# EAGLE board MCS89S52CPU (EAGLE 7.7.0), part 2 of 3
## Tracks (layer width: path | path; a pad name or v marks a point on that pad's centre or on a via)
/CSEX  (via drill 0.61)
  Top 0.254: IC10.1 11.89,57.15 15.54,53.49 v18.06,53.49 | v31.09,50.75 31.09,49.38 v31.77,48.69 31.77,47.78 29.26,45.26 29.26,37.95 31.32,35.89 31.77,35.89 37.95,29.72 v40.23,29.72 | v34.98,50.98 34.98,55.32 40.46,60.81 IC14.20 | v118.87,15.09 117.73,13.95 v115.21,13.95 | v102.87,10.29 101.5,10.29 97.84,6.63 96.01,6.63 95.1,7.54 v95.1,10.29 | v88.01,12.8 86.64,14.17 83.21,14.17 75.44,21.95 75.44,23.32 74.52,24.23 72.69,24.23 v71.09,25.83 | v59.66,29.03 55.78,29.03 55.09,29.72 v43.2,29.72
  Bottom 0.254: v18.06,53.49 23.09,53.49 24.69,51.89 29.95,51.89 v31.09,50.75 | v31.77,48.69 32.69,48.69 v34.98,50.98 | v118.87,15.09 124.36,15.09 IC4.8 | v115.21,13.95 111.56,10.29 v102.87,10.29 | v95.1,10.29 90.53,10.29 v88.01,12.8 | v71.09,25.83 70.41,25.83 67.21,29.03 v59.66,29.03 | v40.23,29.72 v43.2,29.72
ADR0  (via drill 0.61)
  Top 0.254: v90.3,77.04 88.01,77.04 85.95,74.98 v82.07,74.98 | v71.55,68.58 71.55,64.69 72.01,64.24 72.01,61.95 68.58,58.52 IC2.10 | SV1.9 28.12,97.61 28.12,95.33 SV3.9 28.12,95.1 28.12,83.9 v30.86,81.15 | 39.09,56.46 40.01,57.38 45.95,57.38 IC3.10 | 39.09,56.46 v36.58,53.95 | v26.52,18.29 26.52,12.8 IC11.9 | v14.4,41.38 14.4,42.06 15.32,42.98 17.83,42.98 20.8,45.95 20.8,54.18 24.92,58.29 25.38,58.29 IC14.10 | v34.52,77.5 34.52,68.12 38.86,63.78 38.86,62.87 37.95,61.95 v37.26,61.95 | 39.09,56.46 v38.41,57.15
  Bottom 0.254: IC8.19 90.3,78.87 v90.3,77.04 | v82.07,74.98 78.41,71.32 77.95,71.32 76.35,69.72 72.69,69.72 v71.55,68.58 | v36.58,53.95 34.75,53.95 33.6,55.09 30.18,55.09 29.95,54.86 24.23,54.86 23.55,55.55 23.55,56.46 25.38,58.29 IC14.10 | v26.52,18.29 18.06,26.75 18.06,30.63 14.4,34.29 v14.4,41.38 | v34.52,77.5 v30.86,81.15 | v37.26,61.95 37.26,61.49 38.63,60.12 38.63,59.21 38.41,58.98 v38.41,57.15 | IC2.10 68.58,58.29 63.78,58.29 62.64,57.15 57.38,57.15 56.24,58.29 47.09,58.29 IC3.10
ADR1  (via drill 0.61)
  Top 0.254: v89.38,72.69 89.38,64.01 89.84,63.55 89.84,62.64 86.87,59.66 v81.38,59.66 | SV1.10 30.63,97.61 30.63,95.33 SV3.10 30.4,95.1 v30.4,83.44 | v24.23,18.97 24.23,12.8 IC11.8 | v13.49,40.46 13.49,41.83 15.09,43.43 17.6,43.43 20.34,46.18 20.34,55.78 25.38,60.81 IC14.9 | v28.12,81.15 28.12,66.52 26.29,64.69 24.46,64.69 23.55,63.78 v23.55,62.64 | v44.35,62.87 46.18,61.04 46.86,61.04 IC3.9
  Bottom 0.254: v89.38,72.69 89.38,82.75 92.58,85.95 100.36,85.95 101.5,84.81 101.5,82.75 100.81,82.07 99.9,82.07 98.3,83.67 97.84,83.67 IC8.18 | v81.38,59.66 79.55,59.66 78.87,58.98 77.04,58.98 75.21,60.81 68.58,60.81 | 68.58,60.81 64.92,60.81 63.78,59.66 61.72,59.66 61.27,60.12 49.15,60.12 48.46,60.81 47.09,60.81 IC3.9 | 68.58,60.81 IC2.9 | v24.23,18.97 24.23,19.89 17.6,26.52 17.6,30.4 13.49,34.52 v13.49,40.46 | v28.12,81.15 v30.4,83.44 | v23.55,62.64 25.38,60.81 IC14.9 25.6,60.81 30.63,60.81 31.32,60.12 33.38,60.12 37.95,64.69 41.6,64.69 43.43,62.87 v44.35,62.87
ADR2  (via drill 0.61)
  Top 0.254: v11.2,72.01 11.2,71.32 9.83,69.95 7.77,69.95 7.09,70.64 7.09,79.55 8.69,81.15 IC9.1 | v116.81,77.72 116.81,70.64 113.61,67.44 113.61,66.29 114.07,65.84 114.07,59.89 112.7,58.52 109.04,58.52 108.36,59.21 97.38,59.21 96.24,60.35 v96.24,62.64 | v86.41,66.52 v88.24,66.52 | v37.95,63.32 v34.52,63.32
  Bottom 0.254: v11.2,72.01 11.89,72.01 13.26,70.64 13.26,69.72 15.54,67.44 19.2,67.44 23.09,63.55 25.38,63.55 IC14.8 25.6,63.32 v34.52,63.32 | v116.81,77.72 116.81,80.01 115.9,80.92 98.53,80.92 96.7,82.75 96.7,84.81 97.38,85.5 98.53,85.5 100.13,83.9 IC8.17 | v96.24,62.64 95.1,62.64 93.73,64.01 93.73,65.84 93.04,66.52 v88.24,66.52 | v86.41,66.52 85.04,66.52 84.35,67.21 82.3,67.21 77.95,62.87 69.04,62.87 68.58,63.32 IC2.8 68.58,63.55 67.44,64.69 61.72,64.69 61.49,64.92 49.38,64.92 48.01,63.55 47.09,63.55 IC3.8 46.86,63.32 45.49,61.95 40.01,61.95 38.63,63.32 v37.95,63.32
ADR3  (via drill 0.61)
  Top 0.254: 11.2,76.35 8.91,78.64 IC9.2 | v11.2,74.07 11.2,76.35 | v79.55,76.58 82.98,80.01 84.35,80.01 84.81,80.47 99.21,80.47 102.41,83.67 102.87,83.67 IC8.16 | v66.98,70.41 66.98,69.49 66.75,69.27 66.75,67.89 68.58,66.06 IC2.7 68.58,65.84 66.29,63.55 66.29,56.69 65.61,56.01 v65.61,54.86 | v50.06,51.21 50.29,51.44 50.29,62.18 48.92,63.55 48.92,64.01 47.09,65.84 IC3.7 47.09,66.06 48.69,67.67 48.69,69.27 48.46,69.49 48.46,82.07 47.32,83.21 v40.23,83.21 | v14.86,80.01 11.2,76.35
  Bottom 0.254: v11.2,74.07 15.54,69.72 19.43,69.72 23.09,66.06 25.38,66.06 IC14.7 | v79.55,76.58 79.55,73.61 76.12,70.18 69.49,70.18 69.27,69.95 67.44,69.95 v66.98,70.41 | v50.06,51.21 51.44,51.21 51.89,51.66 61.27,51.66 61.72,52.12 62.87,52.12 v65.61,54.86 | v14.86,80.01 28.35,80.01 30.4,82.07 32.23,82.07 35.2,79.1 36.12,79.1 v40.23,83.21
ADR4  (via drill 0.61)
  Top 0.254: v23.55,72.24 23.55,70.87 25.38,69.04 25.38,68.58 IC14.6 | IC3.6 45.26,68.58 v44.35,69.49 | v85.5,73.61 84.35,72.47 83.44,72.47 80.7,69.72 80.7,67.89 v81.15,67.44 | v71.09,63.78 71.09,66.06 IC2.6 | v58.75,69.49 v56.92,67.67
  Bottom 0.254: v23.55,72.24 22.86,72.24 20.8,74.3 18.06,74.3 17.14,75.21 13.49,75.21 12.57,76.12 8.91,76.12 IC9.3 | v44.35,69.49 41.83,69.49 41.6,69.72 36.58,69.72 35.43,68.58 IC14.6 | v85.5,73.61 88.01,76.12 88.01,85.27 90.07,87.33 102.18,87.33 104.47,85.04 104.47,84.81 105.39,83.9 IC8.15 | v81.15,67.44 78.18,67.44 74.52,63.78 v71.09,63.78 | IC3.6 50.98,68.58 51.89,67.67 v56.92,67.67 | v58.75,69.49 61.27,69.49 61.72,69.95 66.06,69.95 67.44,68.58 IC2.6
ADR5  (via drill 0.61)
  Top 0.254: v86.87,87.78 86.18,87.78 v84.35,85.95 | v71.32,88.92 70.18,90.07 52.35,90.07 v49.61,92.81 | v36.8,90.3 36.8,85.72 29.03,77.95 v29.03,74.75 | v38.41,75.44 36.8,75.44 v36.58,75.67
  Bottom 0.254: IC2.5 68.58,71.32 65.61,71.32 64.47,72.47 61.72,72.47 60.35,71.09 47.09,71.09 IC3.5 46.86,71.32 46.18,71.32 42.29,75.21 38.63,75.21 v38.41,75.44 | IC9.6 8.69,68.58 8.69,69.04 7.09,70.64 7.09,74.07 8,74.98 13.03,74.98 15.77,72.24 22.17,72.24 23.09,71.32 25.38,71.32 IC14.5 v29.03,74.75 29.95,75.67 v36.58,75.67 | v86.87,87.78 103.56,87.78 107.44,83.9 107.9,83.9 IC8.14 | v84.35,85.95 83.67,85.95 82.3,87.33 76.12,87.33 72.69,90.75 71.78,90.75 71.32,90.3 v71.32,88.92 | v49.61,92.81 49.61,92.13 47.32,89.84 37.26,89.84 v36.8,90.3
ADR6  (via drill 0.61)
  Top 0.254: 11.66,68.81 14.86,72.01 14.86,74.3 15.77,75.21 v19.2,75.21 | v128.7,86.18 v123.67,86.18 | v122.99,36.8 113.39,36.8 108.36,41.83 104.01,41.83 100.36,38.18 v95.78,38.18 | v84.35,42.98 80.92,42.98 79.78,41.83 v78.87,41.83 | v72.69,47.09 61.72,47.09 56.01,52.81 56.01,56.69 | 56.01,56.69 56.01,69.27 57.61,70.87 | 57.61,70.87 61.72,74.98 67.44,74.98 68.58,73.84 IC2.4 | 57.61,70.87 v56.46,72.01 | v13.72,66.75 11.66,68.81 | 56.01,56.69 v56.46,56.69 | 11.66,68.81 v11.43,68.58
  Bottom 0.254: v11.43,68.58 11.43,57.61 8.91,55.09 8.91,54.63 IC10.2 | v19.2,75.21 24,75.21 25.38,73.84 IC14.4 | v123.67,86.18 122.99,86.87 113.16,86.87 110.64,84.35 110.64,83.9 IC8.13 | v128.7,86.18 131.44,86.18 137.16,80.47 152.93,80.47 154.99,78.41 154.99,72.01 155.45,71.55 155.45,46.41 149.73,40.69 149.73,37.72 144.47,32.46 126.64,32.46 122.99,36.12 v122.99,36.8 | v95.78,38.18 94.87,37.26 90.07,37.26 v84.35,42.98 | v78.87,41.83 77.95,41.83 v72.69,47.09 | v56.46,72.01 52.12,72.01 50.52,73.61 47.09,73.61 IC3.4 | v13.72,66.75 13.72,62.18 18.29,57.61 18.29,56.69 18.06,56.46 18.06,55.55 18.52,55.09 19.89,55.09 24.23,59.44 30.63,59.44 34.75,55.32 39.09,55.32 39.55,54.86 44.12,54.86 46.41,57.15 56.01,57.15 v56.46,56.69
ADR7  (via drill 0.61)
  Top 0.254: v45.72,79.78 45.72,78.18 46.86,77.04 46.86,76.35 IC3.3 | v126.87,73.61 v124.13,76.35 | v126.87,66.98 131.9,61.95 131.9,59.89 127.1,55.09 v119.1,55.09 | v114.53,31.55 113.84,31.55 110.87,28.57 110.87,24.92 109.96,24 108.13,24 107.21,23.09 v107.21,21.95 | v52.12,17.83 v59.66,17.83 | v11.66,45.72 11.66,46.63 8.91,49.38 IC10.4
  Bottom 0.254: IC2.3 68.58,76.81 62.87,82.53 61.04,82.53 56.92,78.41 55.55,78.41 53.95,80.01 46.41,80.01 46.18,79.78 v45.72,79.78 39.09,86.41 39.09,87.1 38.18,88.01 21.03,88.01 13.95,80.92 13.95,77.27 | 13.95,77.27 24.46,77.27 25.38,76.35 IC14.3 | 13.95,77.27 7.77,77.27 5.03,74.52 5.03,67.67 7.77,64.92 9.6,64.92 10.74,63.78 10.74,63.09 7.09,59.44 7.09,51.66 8.69,50.06 8.69,49.61 IC10.4 | v124.13,76.35 124.13,79.32 119.56,83.9 118.42,83.9 116.36,85.95 114.76,85.95 113.16,84.35 113.16,83.9 IC8.12 | v126.87,66.98 v126.87,73.61 | v119.1,55.09 119.1,44.58 114.53,40.01 v114.53,31.55 | v107.21,21.95 105.39,21.95 102.41,18.97 97.38,18.97 94.64,16.23 84.81,16.23 78.87,10.29 75.21,10.29 69.27,16.23 64.24,16.23 62.64,17.83 v59.66,17.83 | v52.12,17.83 51.66,17.83 50.06,16.23 25.6,16.23 21.03,20.8 21.03,21.26 15.09,27.2 15.09,32.23 11.66,35.66 v11.66,45.72
ADR8  (via drill 0.61)
  Top 0.254: SV3.13 38.18,95.33 38.18,97.61 SV1.13 | v18.97,56.01 19.43,55.55 19.43,50.29 17.6,48.46 15.77,48.46 11.89,44.58 8.91,44.58 IC10.6 | v37.72,59.66 37.72,60.12 40.01,62.41 41.83,62.41 42.29,62.87 v42.29,67.21 42.29,72.01 IC14.25 40.69,73.84 42.52,75.67 v42.52,80.47 | v58.29,67.67 59.66,69.04 59.66,70.41 62.18,72.92 62.18,73.61 IC3.25 | v38.18,86.64 38.18,87.55 | 38.18,87.55 v38.18,90.75 | v80.92,92.35 76.81,92.35 72.01,87.55 67.89,87.55 67.44,88.01 53.26,88.01 v52.81,87.55 | 38.18,87.55 v40.01,87.55
  Bottom 0.254: IC1.21 140.82,61.04 135.79,66.06 116.59,66.06 112.7,69.95 87.55,69.95 83.9,73.61 IC2.25 83.9,73.84 83.9,74.52 87.55,78.18 87.55,85.72 v80.92,92.35 | v18.97,56.01 20.12,56.01 24,59.89 30.86,59.89 31.09,59.66 v37.72,59.66 | v58.29,67.67 57.38,66.75 48.01,66.75 47.55,67.21 v42.29,67.21 | v38.18,90.75 38.18,95.1 SV3.13 | v38.18,86.64 42.52,82.3 v42.52,80.47 | v52.81,87.55 50.29,87.55 49.84,88.01 40.46,88.01 v40.01,87.55
ADR9  (via drill 0.61)
  Top 0.254: v126.64,56.92 103.56,56.92 v102.64,56.01 | v95.78,50.98 v97.61,50.98 | v88.7,53.26 88.7,54.86 90.3,56.46 90.3,58.29 89.84,58.75 89.84,61.27 90.75,62.18 90.75,66.29 92.58,68.12 92.58,71.55 90.53,73.61 86.87,73.61 84.58,71.32 83.9,71.32 IC2.24 | SV1.14 40.69,97.61 40.69,95.33 SV3.14 40.69,95.1 40.69,91.9 v45.49,87.1 | v22.63,54.41 21.26,53.03 21.26,44.58 17.6,40.92 15.77,40.92 14.4,39.55 8.91,39.55 IC10.8 | v30.63,54.18 30.63,65.15 31.77,66.29 v31.77,69.49 | v60.12,67.67 60.12,69.04 62.18,71.09 IC3.24 | v45.26,81.61 45.26,80.7 44.35,79.78 v44.35,70.87 45.26,69.95 47.32,69.95 48.23,69.04 48.23,68.12 47.32,67.21 46.41,67.21 v45.26,66.06 46.63,64.69 47.55,64.69 48.23,64.01 48.23,63.55 48.69,63.09 v48.69,50.75 | v89.61,45.03 89.61,37.72 87.55,35.66 87.55,34.98 82.98,30.4 77.5,30.4 v75.67,28.57 | v48.23,38.18 46.18,38.18 v45.72,38.63
  Bottom 0.254: v126.64,56.92 129.39,59.66 129.39,61.72 130.3,62.64 136.7,62.64 138.3,61.04 IC1.22 | v97.61,50.98 v102.64,56.01 | 94.87,50.98 v95.78,50.98 | 94.87,50.98 94.41,51.44 90.98,51.44 89.15,53.26 v88.7,53.26 | v22.63,54.41 30.4,54.41 v30.63,54.18 | v31.77,69.49 35.66,69.49 37.26,71.09 40.46,71.09 IC14.24 40.69,71.09 40.92,70.87 v44.35,70.87 | v60.12,67.67 57.84,65.38 48.01,65.38 47.32,64.69 46.63,64.69 v45.26,66.06 | v45.49,87.1 45.49,81.84 v45.26,81.61 | 94.87,50.98 94.87,50.06 92.81,48.01 92.13,48.01 89.61,45.49 v89.61,45.03 | v75.67,28.57 75.21,28.57 74.3,29.49 72.47,29.49 67.67,34.29 52.12,34.29 v48.23,38.18 | v45.72,38.63 45.72,48.69 46.63,49.61 47.55,49.61 v48.69,50.75
ADR10  (via drill 0.61)
  Top 0.254: IC14.21 40.46,63.32 40.01,63.32 34.06,57.38 v34.06,43.66 34.06,43.2 34.98,42.29 36.58,42.29 40.23,45.95 48.69,45.95 50.29,47.55 v50.29,48.69 | SV1.15 43.2,97.61 43.2,95.33 SV3.15 43.2,95.1 43.2,92.81 47.32,88.7 47.32,84.58 49.84,82.07 49.84,75.89 50.29,75.44 50.29,64.24 v50.06,64.01 | v95.78,54.63 96.24,54.18 126.87,54.18 132.36,59.66 132.36,62.18 132.82,62.64 134.19,62.64 135.79,61.04 IC1.23 | v52.35,63.09 v52.35,50.75
  Bottom 0.254: IC10.11 23.77,34.29 31.77,42.29 32.69,42.29 v34.06,43.66 | v95.78,54.63 92.58,54.63 91.44,53.49 90.53,53.49 85.5,58.52 85.5,61.72 83.9,63.32 IC2.21 83.67,63.32 81.15,63.32 80.01,62.18 68.12,62.18 66.98,63.32 62.41,63.32 IC3.21 61.72,64.01 52.35,64.01 | 52.35,64.01 v50.06,64.01 | v52.35,50.75 v50.29,48.69 | 52.35,64.01 v52.35,63.09
ADR11  (via drill 0.61)
  Top 0.254: v28.35,40.69 28.35,41.38 28.8,41.83 28.8,45.49 30.18,46.86 30.18,52.35 31.77,53.95 v31.77,61.04 | SV1.16 SV3.16 45.72,95.1 51.89,88.92 v69.95,88.92 | v114.07,74.52 114.07,76.81 115.9,78.64 120.47,78.64 136.93,62.18 136.93,59.89 136.25,59.21 135.56,59.21 133.96,60.81 133.5,60.81 IC1.24 | v88.01,70.87 86.18,70.87 83.9,68.58 IC2.23 | v74.98,82.3 75.67,82.3 76.81,83.44 v77.27,83.44 | v77.95,75.21 77.95,74.75 77.5,74.3 77.5,69.49 v78.64,68.35
  Bottom 0.254: v28.35,40.69 27.2,39.55 16.69,39.55 IC10.13 | v31.77,61.04 33.6,61.04 38.86,66.29 38.86,66.98 40.46,68.58 IC14.23 44.81,68.58 46.18,69.95 50.29,69.95 51.66,68.58 IC3.23 63.09,68.58 66.52,65.15 67.67,65.15 68.12,64.69 74.75,64.69 78.41,68.35 v78.64,68.35 83.44,68.35 83.67,68.58 IC2.23 | v114.07,74.52 112.93,74.52 109.5,71.09 96.47,71.09 95.78,70.41 88.47,70.41 v88.01,70.87 | v69.95,88.92 69.95,87.33 v74.98,82.3 | v77.27,83.44 77.27,75.89 v77.95,75.21
ADR12  (via drill 0.61)
  Top 0.254: SV3.17 48.23,95.33 48.23,97.61 SV1.17 | 26.52,62.41 24.69,62.41 19.89,57.61 19.89,48.23 16.69,45.03 16.69,44.58 IC10.15 | 26.52,62.41 29.95,65.84 v29.95,76.58 | v124.13,50.98 121.39,50.98 120.47,51.89 95.33,51.89 v93.95,50.52 | v86.87,46.41 85.27,44.81 85.27,40.23 v84.81,39.78 | v73.61,36.8 57.61,36.8 55.09,34.29 v43.66,34.29 | v30.18,33.6 30.18,34.29 26.06,38.41 26.06,42.06 26.98,42.98 26.98,47.55 27.2,47.78 27.2,61.72 26.52,62.41 | IC2.2 68.58,77.95 70.41,76.12 v70.41,72.24 | v47.78,91.67 47.78,84.81 50.75,81.84 v50.75,79.1
  Bottom 0.254: IC14.2 25.6,78.64 27.66,76.58 v29.95,76.58 34.98,76.58 38.18,79.78 41.83,79.78 42.75,78.87 46.86,78.87 IC3.2 47.78,77.95 50.75,77.95 | v124.13,50.98 130.76,57.61 130.76,60.81 IC1.25 | v93.95,50.52 91.9,48.46 88.92,48.46 v86.87,46.41 | v84.81,39.78 84.81,39.32 85.5,38.63 85.5,37.72 85.04,37.26 74.07,37.26 v73.61,36.8 | v43.66,34.29 43.66,36.35 37.72,42.29 36.58,42.29 30.18,35.89 v30.18,33.6 | v70.41,72.24 69.27,72.24 69.04,72.47 65.15,72.47 63.55,74.07 63.55,79.1 62.64,80.01 59.21,80.01 57.15,77.95 50.75,77.95 | v47.78,91.67 48.23,92.13 48.23,95.1 SV3.17 | 50.75,77.95 v50.75,79.1
ADR13  (via drill 0.61)
  Top 0.254: v114.53,66.75 114.53,59.89 116.13,58.29 125.27,58.29 127.79,60.81 128.25,60.81 IC1.26 | SV1.18 50.98,97.61 50.98,95.33 SV3.18 50.98,95.1 v53.03,93.04 | v22.63,67.89 22.63,61.04 18.06,56.46 18.06,55.55 18.97,54.63 18.97,52.35 16.69,50.06 16.69,49.61 IC10.17 | v38.41,74.07 40.46,76.12 IC14.26 | 62.87,82.53 63.55,81.84 63.55,78.18 62.41,77.04 62.41,76.35 IC3.26 | 62.87,82.53 55.78,82.53 53.26,80.01 53.26,65.38 51.44,63.55 51.44,49.61 52.12,48.92 52.12,47.09 49.15,44.12 | 49.15,44.12 45.03,40.01 32.23,40.01 31.32,40.92 31.32,42.29 v32.23,43.2 | v63.55,93.04 68.12,93.04 v69.72,91.44 | v66.98,87.1 65.61,87.1 65.15,87.55 64.24,87.55 62.87,86.18 62.87,82.53 | v91.21,59.44 91.21,56.01 90.07,54.86 90.07,52.58 87.1,49.61 v87.1,48.92 | v73.61,50.06 72.92,50.06 70.87,52.12 68.12,52.12 64.24,48.23 v64.24,48.01 | 49.15,44.12 v49.84,44.12
  Bottom 0.254: v114.53,66.75 111.33,66.75 111.1,66.98 100.36,66.98 98.98,65.61 98.98,63.78 98.3,63.09 97.38,63.09 96.24,64.24 96.24,66.06 94.41,67.89 87.78,67.89 | 87.78,67.89 85.04,70.64 85.04,71.78 84.35,72.47 83.21,72.47 82.53,73.15 82.53,74.07 83.67,75.21 83.67,76.12 IC2.26 | v22.63,67.89 24.46,69.72 28.57,69.72 29.26,69.04 30.18,69.04 30.86,69.72 30.86,70.41 34.52,74.07 v38.41,74.07 | v32.23,43.2 32.23,43.66 26.52,49.38 16.69,49.38 IC10.17 | v63.55,93.04 v53.03,93.04 | v69.72,91.44 69.72,90.75 66.98,88.01 v66.98,87.1 | 87.78,67.89 87.78,67.44 87.33,66.98 87.33,63.32 v91.21,59.44 | v87.1,48.92 85.04,48.92 84.35,49.61 82.98,49.61 82.07,50.52 74.07,50.52 v73.61,50.06 | v64.24,48.01 63.78,48.01 61.49,45.72 51.44,45.72 v49.84,44.12
ADR14  (via drill 0.61)
  Top 0.254: SV3.19 53.49,95.33 53.49,97.61 SV1.19 | v49.38,87.1 49.38,90.07 v49.15,90.3 | 118.64,30.86 117.04,32.46 114.07,32.46 109.73,28.12 109.27,28.12 IC6.13 | 118.64,30.86 119.79,29.72 119.79,13.03 121.39,11.43 122.3,11.43 123.22,12.34 123.22,13.03 122.76,13.49 122.76,16 124.36,17.6 IC4.9 | 118.64,30.86 v122.07,34.29 | v87.1,61.27 86.87,61.04 83.9,61.04 IC2.20 | v96.24,58.52 108.36,58.52 109.04,57.84 127.33,57.84 129.39,59.89 129.39,61.95 128.7,62.64 127.33,62.64 125.73,61.04 IC1.27 | v64.69,86.64 66.06,86.64 67.44,85.27 68.58,85.27 72.47,81.38 v72.47,58.52
  Bottom 0.254: v49.15,90.3 49.15,90.98 53.26,95.1 SV3.19 | IC3.1 47.09,81.38 47.09,84.81 v49.38,87.1 51.89,87.1 52.35,86.64 v64.69,86.64 | IC1.27 125.73,53.95 123.22,51.44 123.22,50.52 126.87,46.86 126.87,42.29 122.07,37.49 v122.07,34.29 | v87.1,61.27 88.01,61.27 90.75,58.52 v96.24,58.52 | v72.47,58.52 76.12,58.52 76.58,58.06 82.3,58.06 83.21,57.15 84.35,57.15 85.04,57.84 85.04,59.66 83.9,60.81 IC2.20
ADR15  (via drill 0.61)
  Top 0.254: SV1.20 56.01,97.61 56.01,95.33 SV3.20 56.01,95.1 58.52,95.1 63.09,90.53 71.55,90.53 v72.24,89.84 | v64.92,74.07 64.92,72.01 62.87,69.95 61.72,69.95 61.04,69.27 61.04,62.87 62.18,61.72 62.18,61.04 IC3.20 | v64.92,79.1 64.92,82.3 67.44,84.81 68.35,84.81 68.81,84.35 68.81,81.61 68.58,81.38 IC2.1 | v122.07,27.43 122.07,22.63 124.36,20.34 IC4.10 | v107.9,34.29 107.67,34.52 95.78,34.52 95.33,34.06 95.33,33.15 95.78,32.69 95.78,30.18 94.18,28.57 94.18,28.12 IC5.13 | v74.75,78.18 74.75,72.01 75.21,71.55 75.21,48.23 v72.47,45.49 | v77.04,41.15 80.7,37.49 v80.7,34.29
  Bottom 0.254: v64.92,79.1 v64.92,74.07 | v72.24,89.84 72.24,86.41 75.89,82.75 75.89,81.15 74.75,80.01 | 74.75,80.01 69.72,80.01 68.58,81.15 IC2.1 | 81.15,33.83 81.38,34.06 88.01,34.06 93.95,28.12 IC5.13 | 81.15,33.83 80.7,33.38 80.7,32.69 81.15,32.23 81.15,21.03 77.95,17.83 73.84,17.83 IC7.9 | 121.16,29.49 121.16,28.35 v122.07,27.43 | 121.16,29.49 121.16,37.26 124.36,40.46 124.36,46.63 122.76,48.23 122.76,51.66 122.99,51.89 122.99,60.81 IC1.28 | v107.9,34.29 110.41,34.29 115.21,29.49 121.16,29.49 | v74.75,78.18 74.75,80.01 | v72.47,45.49 72.47,43.89 75.21,41.15 v77.04,41.15 | 81.15,33.83 v80.7,34.29
ALE
  Bottom 0.254: IC4.1 116.81,30.63 116.81,41.6 119.56,44.35 119.56,54.18 120.47,55.09 120.47,56.92 118.19,59.21 118.19,60.81 IC1.30
ALE-DISABLE
  Top 0.254: IC1.4 100.36,45.72 100.36,40.69 R2.2
  Bottom 0.254: IC4.2 116.81,28.12 111.33,28.12 109.96,29.49 107.21,29.49 104.01,32.69 104.01,36.8 100.36,40.46 R2.2
ALE-OUT  (via drill 0.61)
  Top 0.254: SV4.10 87.78,95.33 87.78,97.61 SV2.10 | v134.42,25.6 134.42,26.29 139.9,31.77 139.9,34.98 142.19,37.26 142.19,41.15 141.5,41.83 v134.65,41.83 | v130.76,76.35 v133.5,73.61 | v127.1,76.35 125.96,76.35 120.93,81.38 v119.79,81.38 | v103.56,88.92 106.76,88.92 110.19,85.5 113.84,85.5 115.44,83.9 IC8.11
  Bottom 0.254: v134.42,25.6 130.53,21.72 123.67,21.72 119.79,17.83 117.04,17.83 IC4.6 | v134.65,41.83 134.65,51.66 142.42,59.44 142.42,64.69 v133.5,73.61 | v127.1,76.35 v130.76,76.35 | v119.79,81.38 118.19,82.98 116.36,82.98 115.67,83.67 IC8.11 | v103.56,88.92 94.41,88.92 88.24,95.1 87.78,95.1 SV4.10
C02CH  (via drill 0.61)
  Top 0.254: SV3.4 15.32,95.33 15.32,97.61 SV1.4 | v22.86,69.49 22.86,69.04 24.46,67.44 26.52,67.44 27.2,68.12 v27.2,90.3
  Bottom 0.254: v22.86,69.49 21.26,71.09 16.69,71.09 IC9.12 | v27.2,90.3 20.12,90.3 15.32,95.1 SV3.4
C03CH
  Top 0.254: IC9.7 8.91,65.84 14.63,65.84 15.54,64.92 17.6,64.92 21.49,68.81 21.49,70.64 22.17,71.32 22.17,83.21 25.38,86.41 25.38,95.1 SV3.8 25.38,95.33 25.38,97.61 SV1.8
C020H  (via drill 0.61)
  Top 0.254: v11.66,70.18 12.12,70.64 12.12,74.3 16.46,78.64 IC9.15 | v12.34,53.26 9.6,50.52 7.77,50.52 7.09,49.84 v7.09,42.75 | v17.37,17.83 17.37,14.4 18.97,12.8 IC11.6
  Bottom 0.254: v11.66,70.18 11.66,69.72 12.34,69.04 v12.34,53.26 | v7.09,42.75 7.09,41.6 8.23,40.46 10.06,40.46 10.74,39.78 10.74,29.49 10.29,29.03 10.29,24.92 v17.37,17.83
C024H
  Top 0.254: SV1.2 10.29,97.61 10.29,95.33 SV3.2 10.29,95.1 12.34,93.04 14.86,93.04 18.29,89.61 18.29,78.41 16.69,76.81 16.69,76.35 IC9.14
C028H
  Top 0.254: SV1.3 12.8,97.61 12.8,95.33 SV3.3 12.8,95.1 14.4,93.5 15.09,93.5 20.12,88.47 20.12,74.75 19.2,73.84 16.69,73.84 IC9.13
C030H
  Top 0.254: IC9.11 16.69,68.58 16.69,69.04 20.8,73.15 20.8,92.13 17.83,95.1 SV3.5 17.83,95.33 17.83,97.61 SV1.5
C034H
  Top 0.254: IC9.10 16.69,66.06 16.69,66.52 21.49,71.32 21.49,93.95 20.34,95.1 SV3.6 20.34,95.33 20.34,97.61 SV1.6
C038H  (via drill 0.61)
  Top 0.254: v26.29,91.67 26.29,86.64 22.63,82.98 22.63,71.09 21.95,70.41 21.95,68.58 17.83,64.47 17.6,64.47 16.69,63.55 IC9.9 | SV3.7 SV1.7
  Bottom 0.254: v26.29,91.67 22.86,95.1 SV3.7
CLOCK  (via drill 0.61)
  Top 0.254: SV4.15 100.36,95.33 100.36,97.61 SV2.15 | v124.13,83.44 v127.1,80.47
  Bottom 0.254: v127.1,80.47 136.25,80.47 137.85,78.87 138.3,78.87 IC12.3 | v124.13,83.44 121.61,83.44 120.7,84.35 118.64,84.35 116.59,86.41 113.39,86.41 111.56,84.58 111.56,82.75 110.87,82.07 109.96,82.07 109.5,82.53 109.5,85.95 100.36,95.1 SV4.15
CONSOLE-INPUT  (via drill 0.61)
  Top 0.254: SV2.16 SV4.16 | v106.53,5.26 108.81,5.26 v109.27,5.71 | v121.61,7.54 121.61,10.06 126.19,14.63 126.19,31.09 | v126.19,34.29 126.19,31.09 | v124.59,38.41 123.9,38.41 120.02,42.29 118.64,42.29 115.67,45.26 115.67,45.72 IC1.10 | v129.39,87.33 v124.36,87.33 | 126.19,31.09 v126.42,31.09
  Bottom 0.254: v106.53,5.26 105.61,4.34 105.61,2.74 SV8.18 | v109.27,5.71 119.79,5.71 v121.61,7.54 | v126.19,34.29 126.19,36.8 v124.59,38.41 | v124.36,87.33 111.1,87.33 103.33,95.1 102.87,95.1 SV4.16 | v129.39,87.33 132.13,87.33 132.82,88.01 141.5,88.01 141.96,87.55 141.96,85.72 146.76,80.92 154.08,80.92 154.99,80.01 156.59,80.01 157.5,79.1 157.5,42.98 151.1,36.58 149.96,36.58 144.93,31.55 126.87,31.55 v126.42,31.09
CONSOLE-OUTPUT  (via drill 0.61)
  Top 0.254: SV4.17 105.39,95.33 105.39,97.61 SV2.17 | v108.81,11.2 v102.87,5.26 | v110.64,13.03 110.64,14.4 112.7,16.46 v112.7,29.03 | v111.33,32 111.33,33.83 112.01,34.52 120.02,34.52 v120.24,34.29 | v120.24,43.66 118.19,45.72 IC1.11 | v119.33,88.24 119.33,84.12 126.19,77.27 127.56,77.27 128.25,76.58 v128.25,72.69 | v129.84,47.55 125.27,47.55 124.36,46.63 124.36,44.81 v123.22,43.66
  Bottom 0.254: v102.87,5.26 SV8.17 | v110.64,13.03 v108.81,11.2 | v112.7,29.03 112.7,30.63 v111.33,32 | v120.24,34.29 120.24,39.78 120.7,40.23 120.7,43.2 | v120.24,43.66 120.7,43.2 | v119.33,88.24 112.47,88.24 105.61,95.1 SV4.17 | v128.25,72.69 131.44,72.69 141.96,62.18 141.96,59.66 v129.84,47.55 | v123.22,43.66 121.16,43.66 120.7,43.2
DB0  (via drill 0.61)
  Top 0.254: IC11.34 21.72,28.12 21.72,52.12 25.38,55.78 IC14.11 | IC1.39 95.33,61.04 95.33,64.69 RN1.2 95.33,64.92 95.33,66.52 | 95.33,66.52 95.33,76.12 IC8.2 | SV4.2 67.44,95.33 67.44,97.61 SV2.2 | v71.32,77.72 71.32,71.78 69.49,69.95 68.12,69.95 67.21,69.04 67.21,68.12 68.12,67.21 69.27,67.21 69.95,66.52 69.95,60.58 69.04,59.66 68.12,59.66 67.21,58.75 67.21,57.38 68.58,56.01 IC2.11 | 95.33,66.52 92.35,66.52 91.21,65.38 91.21,60.81 90.3,59.89 90.3,58.98 90.75,58.52 90.75,56.24 89.61,55.09 89.61,52.81 85.04,48.23 85.04,47.78 80.01,42.75 78.87,42.75 78.41,43.2 78.41,51.44 v78.87,51.89
  Bottom 0.254: 68.58,55.78 65.15,55.78 64.01,54.63 61.72,54.63 60.58,55.78 47.09,55.78 IC3.11 46.86,55.78 45.49,54.41 39.32,54.41 38.86,54.86 34.52,54.86 33.6,55.78 25.6,55.78 IC14.11 | v71.32,77.72 69.04,80.01 67.67,80.01 65.61,82.07 65.61,89.38 67.21,90.98 67.21,95.1 SV4.2 | v78.87,51.89 72.47,51.89 68.58,55.78 | 68.58,55.78 IC2.11
DB1  (via drill 0.61)
  Top 0.254: IC1.38 97.84,61.04 97.84,64.69 RN1.3 97.84,64.92 97.84,76.12 IC8.3 97.61,76.35 95.33,78.64 v85.72,78.64 | SV2.3 69.95,97.61 69.95,95.33 SV4.3 69.95,95.1 v73.61,91.44 | IC11.33 24,28.12 24,33.6 23.09,34.52 23.09,50.98 25.38,53.26 IC14.12 | v57.15,53.03 58.29,51.89 | 58.29,51.89 60.58,49.61 62.87,49.61 66.52,53.26 68.58,53.26 IC2.12 | v75.44,89.61 75.44,88.7 v74.3,87.55 | v66.52,73.38 66.52,72.01 65.15,70.64 65.15,56.92 62.87,54.63 61.04,54.63 58.29,51.89 | v79.55,80.01 v81.38,80.01
  Bottom 0.254: IC14.12 25.6,53.26 26.52,52.35 44.81,52.35 45.72,53.26 46.86,53.26 IC3.12 47.09,53.26 47.32,53.03 v57.15,53.03 | v75.44,89.61 v73.61,91.44 | v74.3,87.55 74.3,85.04 75.89,83.44 | 75.89,83.44 76.35,82.98 76.35,78.41 72.92,74.98 68.12,74.98 v66.52,73.38 | v85.72,78.64 84.35,80.01 v81.38,80.01 | v79.55,80.01 79.55,82.53 77.72,84.35 76.81,84.35 75.89,83.44
DB2  (via drill 0.61)
  Top 0.254: IC14.13 25.38,50.75 23.55,48.92 23.55,34.75 26.52,31.77 26.52,28.12 IC11.32 | v37.03,41.38 v38.63,42.98 | IC1.37 100.36,61.04 100.36,64.69 RN1.4 100.36,64.92 100.36,76.12 IC8.4 100.13,76.35 96.93,79.55 v86.64,79.55 | SV4.4 72.47,95.33 72.47,97.61 SV2.4 | 68.58,50.75 71.55,50.75 73.15,49.15 74.07,49.15 74.75,49.84 74.75,71.32 73.84,72.24 73.84,80.47 v74.3,80.92 74.98,80.92 76.58,82.53 v81.38,82.53 | v39.55,39.09 44.81,39.09 47.78,42.06 v50.29,42.06 | 68.58,50.75 v66.52,48.69 | 68.58,50.75 IC2.13
  Bottom 0.254: v38.63,42.98 46.41,50.75 46.86,50.75 IC3.13 | 37.03,39.09 37.03,35.43 30.4,28.8 30.4,26.98 29.72,26.29 28.35,26.29 26.75,27.89 IC11.32 | 37.03,39.09 v37.03,41.38 | v74.3,80.92 71.09,80.92 69.04,82.98 67.44,82.98 66.06,84.35 66.06,89.15 72.24,95.33 SV4.4 | v86.64,79.55 86.64,80.24 84.35,82.53 v81.38,82.53 | v39.55,39.09 37.03,39.09 | v50.29,42.06 59.89,42.06 v66.52,48.69
DB3  (via drill 0.61)
  Top 0.254: IC1.36 RN1.5 IC8.5 | SV2.5 74.98,97.61 74.98,95.33 SV4.5 74.75,95.1 74.75,90.98 71.78,88.01 68.12,88.01 67.67,88.47 52.35,88.47 51.89,88.01 v51.89,83.44 | v48.23,46.86 45.26,46.86 44.81,46.41 42.52,46.41 40.69,48.23 IC14.15 | v79.32,43.66 79.32,43.89 83.67,48.23 IC2.15 83.9,48.46 84.58,48.46 87.33,51.21 87.33,54.18 89.38,56.24 v89.38,56.92 | v56.01,79.32 56.01,72.92 55.55,72.47 55.55,48.69 v56.01,48.23
  Bottom 0.254: IC11.31 29.26,28.12 29.26,37.03 40.46,48.23 IC14.15 | v48.23,46.86 51.66,46.86 53.03,48.23 v56.01,48.23 62.18,48.23 IC3.15 62.41,48.46 63.32,48.46 64.47,49.61 69.04,49.61 69.95,48.69 72.47,48.69 77.5,43.66 v79.32,43.66 | v56.01,79.32 v51.89,83.44 | v89.38,56.92 96.01,56.92 98.98,59.89 98.98,61.72 99.9,62.64 100.36,62.64 102.41,64.69 102.87,64.69 RN1.5
DB4  (via drill 0.61)
  Top 0.254: v28.35,48.92 28.35,48.23 27.43,47.32 27.43,42.75 26.52,41.83 26.52,38.63 31.55,33.6 31.55,28.12 IC11.30 | IC1.35 105.39,61.04 105.39,64.69 RN1.6 105.39,64.92 105.39,76.12 IC8.6 | SV4.6 77.5,95.33 77.5,97.61 SV2.6 | v67.89,83.9 67.89,82.75 67.21,82.07 67.21,75.89 68.12,74.98 69.04,74.98 69.95,74.07 69.95,73.15 69.27,72.47 67.67,72.47 65.61,70.41 65.61,56.69 63.55,54.63 63.55,52.12 IC3.16 62.18,50.98 v60.58,52.58 | v99.9,50.06 94.87,50.06 94.41,49.61 93.5,49.61 92.35,50.75 v90.3,50.75 | v86.41,51.66 84.58,51.66 83.9,50.98 IC2.16
  Bottom 0.254: v28.35,48.92 30.63,48.92 33.6,51.89 39.55,51.89 IC14.16 40.69,50.98 45.49,50.98 46.63,52.12 60.12,52.12 v60.58,52.58 | IC3.16 62.41,50.98 64.47,50.98 68.12,54.63 69.04,54.63 72.69,50.98 83.67,50.98 IC2.16 | v67.89,83.9 67.89,88.24 72.01,92.35 74.52,92.35 77.27,95.1 SV4.6 | v99.9,50.06 105.39,55.55 105.39,60.81 IC1.35 | v90.3,50.75 87.33,50.75 v86.41,51.66
DB5  (via drill 0.61)
  Top 0.254: v40.46,38.18 44.81,38.18 45.72,37.26 48.69,37.26 v50.75,39.32 51.21,39.78 51.21,43.66 50.75,44.12 50.75,45.03 53.26,47.55 v53.26,53.95 | SV2.7 SV4.7 | IC1.34 108.13,61.04 108.13,64.69 RN1.7 108.13,64.92 108.13,76.12 IC8.7 107.9,76.35 104.24,80.01 104.24,84.58 103.33,85.5 99.9,85.5 99.21,84.81 99.21,82.98 98.3,82.07 92.35,82.07 91.9,82.53 v86.64,82.53 | v91.9,49.84 92.58,49.84 93.27,49.15 100.36,49.15 v102.18,50.98 | v76.58,39.78 76.58,40.23 76.12,40.69 76.12,45.72 77.5,47.09 77.5,60.35 77.95,60.81 78.87,60.81 79.78,59.89 79.78,48.23 80.24,47.78 81.15,47.78 82.53,49.15 82.53,52.12 83.67,53.26 IC2.17
  Bottom 0.254: IC11.29 34.29,32 v40.46,38.18 | IC3.17 62.18,53.49 61.72,53.95 v53.26,53.95 52.58,54.63 46.41,54.63 45.26,53.49 40.69,53.49 IC14.17 | v91.9,49.84 86.87,49.84 83.9,52.81 83.9,53.26 IC2.17 | v102.18,50.98 102.18,51.66 107.67,57.15 107.67,60.58 107.9,60.81 IC1.34 | SV4.7 80.01,91.67 86.64,85.04 v86.64,82.53 | v50.75,39.32 73.15,39.32 74.52,40.69 75.67,40.69 v76.58,39.78
DB6  (via drill 0.61)
  Top 0.254: v28.8,53.26 29.26,52.81 29.26,48.46 27.89,47.09 27.89,42.52 26.98,41.6 26.98,38.86 36.8,29.03 36.8,28.12 IC11.28 | v38.41,53.72 40.46,55.78 IC14.18 | SV4.8 82.53,95.33 82.53,97.61 SV2.8 | IC1.33 110.64,61.04 110.64,64.69 RN1.8 110.41,64.92 110.41,76.12 IC8.8 | v89.15,85.04 v89.15,88.7 | v90.3,71.78 90.3,62.41 83.9,56.01 IC2.18 | v57.15,61.04 62.18,56.01 IC3.18
  Bottom 0.254: v28.8,53.26 35.89,53.26 36.12,53.03 37.72,53.03 v38.41,53.72 | IC3.18 62.41,56.01 64.69,56.01 65.84,57.15 72.92,57.15 73.38,57.61 82.07,57.61 83.67,56.01 IC2.18 | v89.15,88.7 82.75,95.1 SV4.8 | v89.15,85.04 89.15,83.21 88.47,82.53 88.47,72.24 88.92,71.78 v90.3,71.78 90.53,71.78 94.18,75.44 94.18,77.27 94.87,77.95 108.81,77.95 110.41,76.35 IC8.8 | v57.15,61.04 56.01,62.18 46.41,62.18 44.12,59.89 40.01,59.89 38.86,58.75 38.86,58.06 40.46,56.46 40.46,56.01 IC14.18
DB7  (via drill 0.61)
  Top 0.254: IC11.27 39.32,28.12 38.86,28.12 31.55,35.43 31.09,35.43 27.43,39.09 27.43,41.15 28.35,42.06 28.35,45.72 29.72,47.09 29.72,64.92 30.86,66.06 30.86,79.1 34.06,82.3 42.06,82.3 43.43,80.92 43.43,61.27 40.69,58.52 IC14.19 | IC1.32 113.16,61.04 113.16,64.69 RN1.9 113.16,64.92 113.16,76.12 IC8.9 | SV2.9 85.27,97.61 85.27,95.33 SV4.9 85.04,95.1 79.1,89.15 77.27,89.15 72.92,84.81 72.92,60.12 v73.38,59.66 | v81.61,49.61 81.61,56.24 83.67,58.29 IC2.19
  Bottom 0.254: IC2.19 83.67,58.52 76.81,58.52 75.67,59.66 v73.38,59.66 64.47,59.66 63.32,58.52 62.41,58.52 IC3.19 62.18,58.52 61.04,59.66 46.41,59.66 45.26,58.52 40.69,58.52 IC14.19 | v81.61,49.61 81.61,48.69 86.18,44.12 90.07,44.12 90.53,44.58 90.53,45.72 92.35,47.55 93.73,47.55 96.7,50.52 96.7,51.44 101.5,56.24 101.5,61.72 102.41,62.64 102.87,62.64 104.01,63.78 104.01,65.61 104.93,66.52 110.87,66.52 112.47,64.92 112.93,64.92 RN1.9
DMA-ACK  (via drill 0.61)
  Top 0.254: SV4.13 95.33,95.33 95.33,97.61 SV2.13 | v119.33,59.44 119.33,63.09 120.93,64.69 v120.93,76.81
  Bottom 0.254: v119.33,59.44 119.33,61.95 118.64,62.64 109.96,62.64 109.5,62.18 109.5,60.35 108.13,58.98 108.13,45.72 IC1.7 | v120.93,76.81 120.93,79.1 121.84,80.01 121.84,80.92 119.33,83.44 118.19,83.44 116.13,85.5 114.99,85.5 114.07,84.58 114.07,82.75 112.93,81.61 109.73,81.61 109.04,82.3 109.04,84.81 100.36,93.5 96.93,93.5 95.33,95.1 SV4.13
EA
  Top 0.254: IC1.31 115.67,61.04 115.67,64.69 RN1.10 115.67,64.92 117.96,64.92 JP1.2
FLASH-OE  (via drill 0.61)
  Top 0.254: v90.3,36.35 88.7,34.75 88.7,20.57 86.41,18.29 86.41,17.83 IC5.6 | v80.7,48.69 80.7,58.98 80.47,59.21 80.47,60.12 80.92,60.58 81.15,60.58 81.61,61.04 v81.61,64.24
  Bottom 0.254: v90.3,36.35 84.58,42.06 83.9,42.06 80.7,45.26 v80.7,48.69 | v81.61,64.24 82.07,64.24 83.67,65.84 IC2.22
FLASH-PROG  (via drill 0.61)
  Top 0.254: JP3.2 82.53,35.66 82.53,39.32 R7.1 82.53,39.55 79.55,39.55 77.95,41.15 77.95,52.35 78.87,53.26 78.87,58.75 78.41,59.21 v78.41,59.89 | v80.7,61.49 80.7,62.87 79.55,64.01 79.55,75.21 82.98,78.64 83.67,78.64 IC2.27
  Bottom 0.254: v80.7,61.49 80.01,61.49 v78.41,59.89
GND
  Top 1.27: IC15.2 142.24,24.13 140.97,25.4 140.97,33.02 142.24,34.29 C16.2
  Bottom 0.254: IC10.12 16.46,37.03 14.86,38.63 14.86,40.23 16.46,41.83 IC10.14 16.46,42.06 14.86,43.66 14.86,46.99 14.86,50.29 16.46,51.89 IC10.18 | IC10.9 8.91,36.8 8.91,34.75 IC10.10 | IC10.7 8.91,42.06 10.74,43.89 10.74,46.99 10.74,50.06 8.91,51.89 IC10.3
  Bottom 1.016: 128.27,11.43 125.73,8.89 116.84,8.89 | 116.84,8.89 107.95,8.89 | 107.95,8.89 101.6,8.89 | 101.6,8.89 97.79,8.89 | 97.79,8.89 86.36,8.89 | 86.36,8.89 74.93,8.89 | 74.93,8.89 66.04,8.89 | 66.04,8.89 63.5,8.89 62.23,10.16 62.23,13.97 60.96,15.24 59.69,15.24 | 59.69,15.24 22.86,15.24 | 22.86,15.24 21.59,13.97 IC11.7 | 1.27,31.75 3.81,34.29 C10.2 IC10.10 | 1.27,31.75 1.27,17.78 2.54,16.51 21.59,16.51 22.86,15.24 | 1.27,63.5 1.27,46.99 | 1.27,46.99 1.27,31.75 | IC9.8 C9.2 1.27,63.5 | C7.2 IC7.7 66.04,8.89 | SV8.6 74.93,8.89 | IC5.7 C5.2 86.36,8.89 | IC6.7 C6.2 101.6,8.89 | SV8.19 107.95,8.89 | SV8.15 97.79,8.89 | IC4.7 C4.2 116.84,8.89 | 59.69,15.24 58.42,16.51 58.42,31.75 C11.1 46.99,40.64 | 46.99,40.64 C3.2 IC3.14 | 46.99,40.64 67.31,40.64 68.58,41.91 C2.2 IC2.14 | C21.1 IC14.14 24.13,48.26 22.86,46.99 IC10.16 14.86,46.99 10.74,46.99 IC10.5 1.27,46.99 | 1.27,63.5 1.27,92.71 2.54,93.98 6.35,93.98 | 6.35,93.98 SV3.1 SV1.1 | IC8.1 92.71,80.01 115.57,80.01 IC8.10 C8.2 118.11,74.93 | 118.11,74.93 JP1.1 | 135.89,34.29 Q2.1 135.89,41.91 137.16,43.18 139.7,43.18 140.97,44.45 IC1.20 C1.2 143.51,46.99 144.78,48.26 151.13,48.26 152.4,49.53 C13.1 C14.1 152.4,73.66 151.13,74.93 | 125.73,74.93 118.11,74.93 | 125.73,74.93 C19.1 125.73,91.44 | 125.73,91.44 125.73,97.79 127,99.06 132.08,99.06 IC13.1 140.97,95.25 142.24,96.52 R1.2 142.24,99.06 144.78,99.06 D3.1 | 125.73,91.44 110.49,91.44 SV4.19 SV2.19 | 6.35,93.98 6.35,91.44 8.89,88.9 64.77,88.9 SV4.1 SV2.1 | IC12.7 C12.2 151.13,74.93 | 151.13,74.93 125.73,74.93
  Bottom 1.27: 140.97,19.05 X1.2 154.94,20.32 D1.A | 140.97,19.05 139.7,20.32 IC15.3 | C16.2 135.89,34.29 C17.2 | C15.2 137.16,3.81 135.89,2.54 129.54,2.54 128.27,3.81 128.27,11.43 135.89,19.05 140.97,19.05 | IC15.4 IC15.3 | IC15.2 IC15.3
  pour Bottom: 1.27,96.52 1.27,99.06 158.75,99.06 158.75,1.27 1.27,1.27
INT0/DMA-REQUEST  (via drill 0.61)
  Top 0.254: SV4.12 92.81,95.33 92.81,97.61 SV2.12 | v114.76,48.69 117.5,48.69 120.47,45.72 IC1.12 | v111.78,59.44 111.78,68.35 111.33,68.81 v111.33,74.3 | v111.56,78.64 110.87,78.64 106.53,82.98 106.53,84.81 103.33,88.01 98.3,88.01 v96.24,90.07
  Bottom 0.254: v114.76,48.69 114.76,49.15 114.99,49.38 114.99,56.24 v111.78,59.44 | v111.33,74.3 111.33,74.75 111.56,74.98 v111.56,78.64 | v96.24,90.07 92.81,93.5 92.81,95.1 SV4.12
INT1  (via drill 0.61)
  Top 0.254: SV2.11 90.3,97.61 90.3,95.33 SV4.11 90.07,95.1 80.47,85.5 76.81,85.5 73.38,82.07 73.38,72.01 74.3,71.09 74.3,58.98 73.84,58.52 v73.84,56.69 | v93.04,52.35 124.13,52.35 125.04,51.44 125.04,50.52 123.22,48.69 123.22,45.72 IC1.13
  Bottom 0.254: v93.04,52.35 90.98,52.35 88.7,54.63 78.87,54.63 76.81,56.69 v73.84,56.69
LINE-PRINTER-OUT  (via drill 0.61)
  Top 0.254: SV2.18 108.13,97.61 108.13,95.33 SV4.18 107.9,95.1 107.44,95.1 105.16,92.81 v104.24,92.81 | v109.27,4.34 102.41,4.34 100.81,2.74 100.36,2.74 SV8.16 | v120.47,4.34 130.76,14.63 130.76,24 138.3,31.55 138.3,39.09 137.62,39.78 136.47,39.78 136.25,39.55 129.84,39.55 127.56,41.83 126.42,41.83 125.73,41.15 125.73,40.23 127.56,38.41 127.79,38.41 128.25,37.95 128.25,37.03 127.79,36.58 125.04,36.58 119.79,41.83 113.39,41.83 110.64,44.58 110.64,45.72 IC1.8 | v110.64,86.41 115.21,86.41 116.81,84.81 116.81,80.47 v117.73,79.55 | v119.79,77.5 119.79,67.89 120.02,67.67 120.02,64.47 118.19,62.64 117.5,62.64 117.04,62.18 v117.04,59.21
  Bottom 0.254: v120.47,4.34 v109.27,4.34 | v110.64,86.41 v104.24,92.81 | v119.79,77.5 v117.73,79.55 | v117.04,59.21 117.04,53.03 115.67,51.66 115.67,48.23 115.21,47.78 114.3,47.78 113.61,48.46 113.61,48.69 113.16,49.15 112.24,49.15 110.64,47.55 110.64,45.72 IC1.8
N$1
  Top 1.27: IC15.7 142.24,16.51 143.51,17.78 146.05,17.78 147.32,19.05 D1.C
  Bottom 1.27: L1.1 148.63,27.98 147.32,26.67 D1.C
N$2
  Top 0.254: IC1.19 138.53,45.72 143.56,50.75 145.85,50.75 Q1.2 146.07,50.75 149.73,50.75 C13.2
N$3
  Bottom 1.27: C15.1 132.08,11.43 133.35,12.7 D2.C 134.62,13.97 135.89,15.24 IC15.5
N$4
  Bottom 1.27: X1.1 149.86,13.97 148.59,12.7 F1.1
N$5
  Bottom 1.27: F1.2 143.51,11.43 D2.A
N$6  (via drill 0.61)
  Top 0.254: IC12.4 141.05,78.87 143.33,78.87 IC12.5 143.56,78.64 v143.56,71.09 | C14.2 149.73,55.78 146.07,55.78 Q1.1
  Bottom 0.254: IC1.18 136.02,45.72 Q1.1 145.85,55.78 143.56,58.06 v143.56,71.09
N$7
  Top 0.254: 136.02,88.7 136.02,88.92 137.16,90.07 R3.2 | 136.02,88.7 136.02,86.41 IC12.13 | 136.02,88.7 132.13,92.58 IC13.3
N$8
  Top 0.254: 116.81,22.86 116.81,20.34 IC4.5 | 116.81,22.86 116.81,25.38 IC4.3 | 116.81,22.86 IC4.4
N$9
  Top 0.254: IC12.1 133.5,78.87 135.79,78.87 IC12.2 137.62,80.47 144.25,80.47 145.85,78.87 IC12.6
N$10
  Top 0.254: IC5.8 94.18,15.32 94.18,15.77 95.78,17.37 95.78,23.77 94.18,25.38 IC5.12
N$11
  Bottom 0.254: IC5.1 86.18,30.4 86.18,29.95 84.58,28.35 84.58,27.43 85.5,26.52 90.3,26.52 93.95,22.86 IC5.11
N$12
  Top 0.254: IC12.12 138.53,86.41 140.13,88.01 146.99,88.01 148.59,86.41 IC12.8
N$13
  Top 0.254: 86.41,22.86 86.41,20.34 IC5.5 | 86.41,22.86 86.41,25.38 IC5.3 | 86.41,22.86 IC5.4
N$14
  Bottom 0.254: IC6.3 101.73,25.6 109.04,25.6 IC6.12
N$15
  Bottom 0.254: IC6.11 IC6.4
N$16
  Top 0.254: IC6.10 109.27,20.12 109.27,17.83 IC6.9
  Bottom 0.254: IC6.6 101.73,17.83 109.04,17.83 IC6.9
N$17
  Top 0.254: 66.06,22.86 66.06,20.34 IC7.5 | 66.06,22.86 66.06,25.38 IC7.3 | 66.06,22.86 IC7.4
N$18
  Top 0.254: R5.1 62.18,24.23 62.18,26.52 C20.2 62.41,26.75 64.69,26.75 65.84,27.89 IC7.2 66.06,28.12 66.06,30.4 IC7.1 66.06,30.63 66.06,35.43 D4.A
N$19
  Bottom 0.254: IC7.6 66.06,17.83 73.61,25.38 IC7.12
N$20
  Top 0.254: IC7.10 73.61,20.34 73.61,22.86 IC7.11
N$21
  Top 0.254: IC7.13 73.84,27.89 74.98,27.89 76.12,26.75 78.64,26.75 JP2.2
N$22
  Top 0.254: JP2.3 78.87,24 78.87,20.34 R6.1
N$23
  Top 0.254: Q2.2 137.16,38.86 128.7,38.86 127.1,40.46 R8.2
N$24
  Bottom 0.254: IC7.8 73.84,15.32 76.12,15.32 82.53,21.72 82.53,32.92 JP3.1
N$25
  Top 0.254: Q2.3 138.53,40.69 140.82,40.69 R9.1
N$26
  Top 0.254: LED1.K 152.25,39.55 149.5,39.55 148.59,40.46 R9.2
N$29
  Top 0.254: IC9.5 8.91,71.32 8.91,73.61 IC9.4
  Bottom 0.254: IC10.19 16.46,54.63 16.46,55.09 12.8,58.75 12.8,70.41 12.12,71.09 8.91,71.09 IC9.5
P10  (via drill 0.61)
  Top 0.254: v77.27,18.75 77.27,17.37 82.53,12.12 82.53,2.74 SV8.9 | v91.9,32.69 91.9,35.66 v94.41,38.18
  Bottom 0.254: v77.27,18.75 77.27,20.57 79.78,23.09 80.01,23.09 80.7,23.77 80.7,32 79.78,32.92 79.78,34.98 81.61,36.8 84.12,36.8 86.41,34.52 89.38,34.52 91.21,32.69 v91.9,32.69 | v94.41,38.18 94.41,44.12 92.81,45.72 IC1.1
P11  (via drill 0.61)
  Top 0.254: v80.47,15.54 84.58,11.43 88.24,11.43 88.92,10.74 88.92,9.83 85.27,6.17 85.27,2.74 SV8.10 | v91.44,24 91.44,25.15 93.04,26.75 94.87,26.75 98.53,30.4 v98.53,32.69
  Bottom 0.254: v80.47,15.54 80.47,16.69 85.5,21.72 89.15,21.72 v91.44,24 | v98.53,32.69 98.53,36.8 95.33,40.01 95.33,45.72 IC1.2
PA0
  Bottom 0.254: SV7.1 11.43,10.06 13.95,12.57 IC11.4
PA1
  Top 0.254: IC11.3 11.43,5.26 13.95,2.74 SV7.2
PA2
  Bottom 0.254: IC11.2 8.91,12.8 9.37,12.8 10.97,14.4 14.4,14.4 15.32,13.49 15.32,3.89 16.46,2.74 SV7.3
PA3
  Bottom 0.254: SV7.4 18.97,2.74 18.97,10.52 17.6,11.89 17.6,13.72 16.46,14.86 8.46,14.86 6.4,12.8 IC11.1
PA4  (via drill 0.61)
  Top 0.254: v15.09,18.75 15.09,11.89 21.49,5.49 21.49,2.74 SV7.5
  Bottom 0.254: v15.09,18.75 15.09,19.2 IC11.40
PA5  (via drill 0.61)
  Top 0.254: v19.89,4.57 12.8,11.66 v12.8,18.97
  Bottom 0.254: v19.89,4.57 21.72,4.57 23.55,2.74 24,2.74 SV7.6 | v12.8,18.97 5.26,26.52 5.26,29.03 5.94,29.72 7.09,29.72 8.69,28.12 IC11.39
PA6  (via drill 0.61)
  Top 0.254: v19.2,18.97 v19.2,15.09
  Bottom 0.254: v19.2,15.09 20.12,14.17 20.12,10.97 26.52,4.57 26.52,2.74 SV7.7 | v19.2,18.97 19.2,20.12 11.43,27.89 IC11.38
PA7  (via drill 0.61)
  Top 0.254: v20.57,18.97 v20.57,15.09
  Bottom 0.254: v20.57,15.09 20.57,11.2 29.03,2.74 SV7.8 | v20.57,18.97 20.57,21.03 14.17,27.43 14.17,27.89 IC11.37
PB0
  Bottom 0.254: SV8.4 69.72,2.74 69.72,3.2 64.92,8 61.49,8 55.09,14.4 51.21,14.4 49.61,12.8 IC11.18
PB1
  Bottom 0.254: SV8.3 67.21,2.74 62.41,7.54 57.15,7.54 52.12,12.57 IC11.19
PB2
  Top 0.254: IC11.20 54.63,12.57 64.69,2.52 SV8.2
PB3  (via drill 0.61)
  Top 0.254: v64.01,4.57 64.01,20.57 56.69,27.89 54.63,27.89 IC11.21
  Bottom 0.254: v64.01,4.57 62.18,2.74 SV8.1
PB4  (via drill 0.61)
  Top 0.254: v52.35,10.52 51.89,10.97 51.66,10.97 50.98,11.66 v50.98,18.52
  Bottom 0.254: v52.35,10.52 59.66,3.2 59.66,2.74 SV7.20 | v50.98,18.52 50.98,26.98 51.89,27.89 IC11.22
PB5
  Top 0.254: SV7.19 57.15,3.66 53.49,7.32 53.49,13.72 54.18,14.4 61.72,14.4 63.55,16.23 63.55,20.34 62.64,21.26 56.24,21.26 49.61,27.89 IC11.23
PB6  (via drill 0.61)
  Top 0.254: v48.23,18.52 48.23,11.89 54.41,5.71 54.41,2.74 SV7.18
  Bottom 0.254: v48.23,18.52 48.23,26.75 47.09,27.89 IC11.24
PB7  (via drill 0.61)
  Top 0.254: v44.58,17.14 44.58,14.86 45.95,13.49 45.95,8.69 51.89,2.74 SV7.17
  Bottom 0.254: v44.58,17.14 44.58,27.89 IC11.25
PC0
  Bottom 0.254: SV7.9 31.77,2.74 31.77,5.03 39.32,12.57 IC11.14
PC1
  Bottom 0.254: SV7.10 34.29,5.03 41.83,12.57 IC11.15
PC2
  Bottom 0.254: SV7.11 37.03,2.74 37.03,5.26 44.35,12.57 IC11.16
PC3
  Bottom 0.254: IC11.17 39.55,5.26 39.55,2.74 SV7.12
PC4
  Top 0.254: IC11.13 37.03,12.57 37.03,7.54 41.83,2.74 SV7.13
PC5
  Top 0.254: IC11.12 34.29,12.8 34.75,12.8 36.35,14.4 37.26,14.4 38.18,13.49 38.18,8.91 44.35,2.74 SV7.14
PC6
  Top 0.254: SV7.15 46.86,2.74 46.86,5.49 40.46,11.89 40.46,13.72 39.32,14.86 33.83,14.86 31.77,12.8 IC11.11
PC7
  Top 0.254: SV7.16 49.38,2.74 49.38,4.57 42.98,10.97 42.98,13.72 41.38,15.32 31.77,15.32 29.26,12.8 IC11.10
PROG-ENABLE
  Top 0.254: 105.39,43.89 100.81,39.32 94.18,39.32 93.5,38.63 93.5,38.18 89.15,33.83 89.15,13.72 89.84,13.03 89.84,12.57 92.58,9.83 92.58,2.74 SV8.13 | 105.39,43.89 105.39,45.72 IC1.6 | 105.39,43.89 106.98,43.89 110.19,40.69 119.33,40.69 R8.1
PROG-PULSE  (via drill 0.61)
  Top 0.254: IC1.5 102.41,45.72 100.58,47.55 v90.3,47.55 | v86.87,45.03 86.87,44.35 85.72,43.2 85.72,39.32 v84.58,38.18 | v78.64,38.18 78.64,33.6 v76.12,31.09 | v63.78,28.12 63.78,30.18 62.41,31.55 C20.1 62.18,31.77 62.18,35.43 R4.1
  Bottom 0.254: v90.3,47.55 89.38,47.55 v86.87,45.03 | v78.64,38.18 v84.58,38.18 | v76.12,31.09 76.12,29.49 76.58,29.03 76.58,28.12 74.98,26.52 72.69,26.52 72.01,25.83 72.01,25.38 71.55,24.92 68.81,24.92 66.98,26.75 65.15,26.75 v63.78,28.12
PSEN
  Top 0.254: IC6.1 101.73,30.4 101.73,28.12 IC6.2
  Bottom 0.254: IC5.2 86.41,27.89 91.9,27.89 93.04,26.75 100.36,26.75 101.5,27.89 IC6.2 | IC1.29 120.47,61.04 120.47,61.49 118.87,63.09 105.39,63.09 104.01,61.72 104.01,55.55 98.98,50.52 98.98,41.6 98.53,41.15 98.53,37.49 101.5,34.52 101.5,30.63 IC6.1
PWM  (via drill 0.61)
  Top 0.254: IC4.12 124.59,25.6 124.59,27.89 IC4.13 | v88.01,7.54 88.01,8.23 89.38,9.6 89.38,12.8 88.7,13.49 88.7,15.09 87.1,16.69 85.27,16.69 84.58,17.37 84.58,31.32 89.38,36.12 89.38,36.8 97.61,45.03 97.61,45.72 IC1.3 | v103.56,16.92 103.56,14.86 104.01,14.4 104.01,13.49 98.07,7.54 v96.47,7.54
  Bottom 0.254: SV8.8 80.01,2.74 80.47,2.74 85.27,7.54 v88.01,7.54 88.47,8 94.87,8 95.33,7.54 v96.47,7.54 | v103.56,16.92 103.78,16.69 110.41,16.69 112.7,18.97 117.96,18.97 124.36,25.38 IC4.12
RAM-OE  (via drill 0.61)
  Top 0.254: v112.47,33.6 112.47,31.55 110.41,29.49 108.58,29.49 106.3,27.2 106.3,18.52 109.04,15.77 109.04,15.32 IC6.8 | v112.93,43.66 111.78,44.81 v111.78,50.98 | v110.64,55.09 96.7,55.09 93.95,57.84 v93.95,59.44 | v88.92,63.09 88.47,63.09 84.35,67.21 83.44,67.21 81.61,69.04 v81.61,69.27 | v64.24,68.81 64.24,67.89 62.41,66.06 IC3.22
  Bottom 0.254: v112.47,33.6 112.47,43.2 v112.93,43.66 | v111.78,50.98 111.78,53.95 v110.64,55.09 | v93.95,59.44 93.95,61.95 92.81,63.09 v88.92,63.09 | v81.61,69.27 73.61,69.27 71.55,67.21 65.84,67.21 v64.24,68.81
RD  (via drill 0.61)
  Top 0.254: SV1.11 33.15,97.61 33.15,95.33 SV3.11 33.15,95.1 35.66,92.58 v35.66,87.1 | v35.66,80.01 35.66,70.87 40.46,66.06 IC14.22 | 45.95,19.43 60.35,19.43 v60.81,18.97 | 45.95,19.43 33.83,19.43 28.12,13.72 28.12,11.89 27.2,10.97 18.29,10.97 16.69,12.57 IC11.5 | IC5.9 93.95,17.83 93.95,20.12 IC5.10 | v142.42,26.06 145.39,29.03 145.39,39.32 141.5,43.2 136.02,43.2 133.5,45.72 IC1.17 | v99.9,16.69 99.9,18.52 101.5,20.12 IC6.5 | v44.58,64.24 46.63,62.18 47.55,62.18 48.23,61.49 48.23,52.81 47.55,52.12 46.63,52.12 44.35,49.84 v44.35,47.32 | 45.95,19.43 v45.95,18.97
  Bottom 0.254: v35.66,87.1 v35.66,80.01 | v60.81,18.97 62.64,18.97 64.92,16.69 69.95,16.69 72.47,14.17 80.47,14.17 85.5,19.2 92.58,19.2 93.5,20.12 93.95,20.12 IC5.10 | IC6.5 101.5,20.12 97.38,20.12 95.1,17.83 94.18,17.83 IC5.9 | v142.42,26.06 136.25,26.06 126.42,16.23 104.24,16.23 104.01,16 103.1,16 102.41,16.69 v99.9,16.69 | v44.58,64.24 42.98,65.84 40.69,65.84 IC14.22 | v44.35,47.32 44.35,34.98 45.72,33.6 45.72,31.32 45.95,31.09 v45.95,18.97
RESET  (via drill 0.61)
  Top 0.254: SV2.14 97.84,97.61 97.84,95.33 SV4.14 97.61,95.1 94.87,92.35 89.38,92.35 v80.47,83.44 | 104.47,33.15 104.47,10.52 103.33,9.37 102.41,9.37 95.78,2.74 95.33,2.74 SV8.14 | v104.93,33.6 104.47,33.15 | v45.03,30.63 46.41,30.63 46.86,30.18 v62.41,30.18 | v71.55,29.03 74.75,29.03 75.89,30.18 76.58,30.18 78.18,31.77 83.67,31.77 86.64,34.75 v86.64,35.66 86.64,43.43 89.38,46.18 89.38,51.21 90.98,52.81 v90.98,54.41 | v96.24,33.6 104.01,33.6 104.47,33.15 | v154.53,71.09 154.08,71.09 147.45,77.72 147.45,79.78 141.05,86.18 IC12.11 | v125.96,38.41 121.61,42.75 118.87,42.75 116.59,45.03 116.59,46.86 115.9,47.55 114.99,47.55 113.16,45.72 IC1.9 | v80.47,74.75 80.47,70.18 80.24,69.95 80.24,66.98 82.53,64.69 84.35,64.69 v86.18,62.87
  Bottom 0.254: v104.93,33.6 104.93,35.89 112.01,42.98 112.01,44.81 112.93,45.72 IC1.9 | v45.03,30.63 42.75,30.63 42.52,30.4 41.6,30.4 41.38,30.63 39.78,30.63 38.18,29.03 38.18,27.2 36.35,25.38 21.72,25.38 19.2,27.89 IC11.35 | v62.41,30.18 64.24,30.18 64.92,29.49 71.09,29.49 v71.55,29.03 | v86.64,35.66 88.92,35.66 90.98,33.6 v96.24,33.6 | v154.53,71.09 154.53,48.23 144.93,38.63 144.93,33.6 144.25,32.92 131.44,32.92 v125.96,38.41 | v80.47,74.75 v80.47,83.44 | v86.18,62.87 86.18,58.75 90.53,54.41 v90.98,54.41
RESET-IN  (via drill 0.61)
  Top 0.254: S1.2 155.91,96.24 155.68,96.01 152.93,96.01 152.48,96.47 D3.2 152.25,96.47 147.22,91.44 | 147.22,91.44 143.56,91.44 142.42,90.3 R1.1 | 147.22,91.44 C18.2 | v76.12,11.2 72.47,7.54 72.47,2.74 SV8.5 | v113.61,20.57 113.61,15.09 112.93,14.4 112.93,10.52 120.02,3.43 120.93,3.43 133.5,16 133.5,26.06 139.45,32 v139.45,35.89 | v153.62,78.41 145.85,86.18 IC12.9 145.85,86.41 143.56,86.41 IC12.10
  Bottom 0.254: v76.12,11.2 79.1,11.2 84.58,16.69 90.75,16.69 93.27,19.2 95.78,19.2 100.58,24 110.19,24 v113.61,20.57 | v139.45,35.89 140.36,35.89 153.62,49.15 v153.62,78.41 | R1.1 142.42,90.07 142.42,87.33 143.33,86.41 IC12.10
T0  (via drill 0.61)
  Top 0.254: v95.1,5.71 93.73,5.71 93.27,6.17 93.27,12.34 97.61,16.69 97.61,23.55 100.81,26.75 102.64,26.75 103.56,27.66 v103.56,31.32 | v112.7,48.23 112.7,49.84 113.61,50.75 120.93,50.75 122.07,49.61 122.07,43.43 122.76,42.75 123.67,42.75 125.73,44.81 IC1.14
  Bottom 0.254: v95.1,5.71 95.1,7.09 94.64,7.54 93.04,7.54 88.24,2.74 87.78,2.74 SV8.11 | v103.56,31.32 103.56,35.66 98.98,40.23 98.98,40.92 101.96,43.89 110.87,43.89 111.56,44.58 111.56,47.09 v112.7,48.23
T1  (via drill 0.61)
  Top 0.254: v94.18,6.63 94.18,10.74 97.38,13.95 v103.1,13.95 | v113.84,13.95 121.16,6.63 122.07,6.63 129.84,14.4 129.84,23.77 134.87,28.8 134.87,37.72 v134.65,37.95
  Bottom 0.254: v94.18,6.63 90.3,2.74 SV8.12 | v113.84,13.95 v103.1,13.95 | v134.65,37.95 134.65,39.32 128.25,45.72 IC1.15
VCC
  Top 1.016: 41.91,20.32 3.81,20.32 1.27,22.86 1.27,39.37 | 1.27,39.37 1.27,59.69 | 1.27,59.69 1.27,68.58 | C17.1 130.81,29.21 129.54,30.48 129.54,34.29 128.27,35.56 124.46,35.56 | 124.46,35.56 109.22,35.56 | 107.95,35.56 95.25,35.56 93.98,34.29 IC5.14 91.44,30.48 90.17,29.21 90.17,13.97 C5.1 | 109.22,35.56 IC6.14 106.68,30.48 105.41,29.21 105.41,13.97 C6.1 109.22,12.7 110.49,11.43 SV8.20 | 124.46,35.56 IC4.14 121.92,30.48 120.65,29.21 120.65,13.97 C4.1 | 109.22,35.56 107.95,35.56 | 107.95,35.56 R2.1 | L1.2 157.44,35.52 158.75,36.83 158.75,41.91 | 158.75,41.91 158.75,53.34 | 158.75,53.34 158.75,69.85 | 113.03,91.44 92.71,91.44 IC8.20 85.09,83.82 83.82,82.55 IC2.28 77.47,81.28 76.2,80.01 76.2,46.99 C2.1 73.66,40.64 R7.2 | 130.81,86.36 129.54,85.09 129.54,71.12 130.81,69.85 158.75,69.85 | IC12.14 130.81,86.36 | 130.81,86.36 C19.2 130.81,90.17 129.54,91.44 125.73,91.44 | 113.03,91.44 SV4.20 SV2.20 | 125.73,91.44 125.73,93.98 | IC13.2 125.73,93.98 | 125.73,93.98 125.73,97.79 127,99.06 135.89,99.06 R3.1 | C9.1 1.27,68.58 | C11.2 41.91,20.32 | 41.91,20.32 62.23,20.32 R5.2 | R4.2 52.07,35.56 | 158.75,53.34 95.25,53.34 92.71,55.88 IC1.40 RN1.1 | 158.75,41.91 LED1.A 152.4,44.45 151.13,45.72 C1.1 | 52.07,35.56 41.91,35.56 | C11.2 IC11.26 | C11.2 41.91,35.56 | 41.91,35.56 40.64,36.83 31.75,36.83 30.48,38.1 C21.2 33.02,45.72 33.02,80.01 34.29,81.28 IC14.28 | 52.07,35.56 52.07,38.1 | 52.07,38.1 C3.1 54.61,46.99 54.61,80.01 55.88,81.28 IC3.28 | C10.1 1.27,39.37 | IC10.20 16.51,58.42 15.24,59.69 1.27,59.69 | 113.03,91.44 118.11,91.44 | 118.11,91.44 125.73,91.44 | 158.75,69.85 158.75,78.74 | 157.48,78.74 C12.1 158.75,78.74
  Top 1.016: 158.75,78.74 158.75,90.42 S1.1 157.2,91.72 156.21,92.71 151.13,92.71 C18.1 | C8.1 118.11,91.44 | SV8.7 77.47,11.43 R6.2 C7.1 69.85,13.97 69.85,29.21 71.12,30.48 IC7.14 73.66,34.29 74.93,35.56 D4.C 74.93,36.83 R7.2 | R7.2 73.66,38.1 52.07,38.1 | 1.27,68.58 1.27,90.17 2.54,91.44 15.24,91.44 16.51,90.17 IC9.16
  Bottom 1.27: L1.2 151.09,35.52 149.86,34.29 149.86,31.75 148.59,30.48 144.78,30.48 C16.1 | IC15.1 144.78,27.94 C16.1 | C16.1 C17.1
  pour Top: 1.27,99.06 158.75,99.06 158.75,20.32 135.89,20.32 127,11.43 127,1.27 1.27,1.27
WR  (via drill 0.61)
  Top 0.254: v142.42,30.63 144.93,33.15 144.93,39.09 141.28,42.75 133.96,42.75 130.99,45.72 IC1.16 | SV1.12 35.66,97.61 35.66,95.33 SV3.12 35.66,95.1 36.12,95.1 49.38,81.84 v49.38,74.98 | v20.8,32.23 IC11.36 | v32.23,41.38 35.66,41.38 36.58,40.46 44.81,40.46 51.21,46.86 v51.21,47.78 51.21,49.15 50.98,49.38 50.98,71.78 v52.35,73.15
  Bottom 0.254: v142.42,30.63 129.39,30.63 125.27,26.52 105.16,26.52 102.18,29.49 100.36,29.49 97.16,32.69 97.16,34.06 95.78,35.43 89.84,35.43 85.72,39.55 85.72,40.23 85.27,40.69 80.24,40.69 | 80.24,40.69 79.32,40.69 76.35,37.72 73.15,37.72 72.69,37.26 72.69,35.89 78.64,29.95 78.64,29.26 JP2.1 | v20.8,32.23 23.09,32.23 v32.23,41.38 | IC3.27 62.18,78.64 56.69,73.15 v52.35,73.15 50.52,74.98 v49.38,74.98 45.95,74.98 42.29,78.64 40.69,78.64 IC14.27 | 80.24,40.69 80.24,44.12 75.21,49.15 72.01,49.15 69.04,52.12 66.29,52.12 63.78,49.61 53.03,49.61 v51.21,47.78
